(* Logix 5000 Rung export; software revision 16.04 *)

MODULES
   Local : vendor None type None code None
   MVI56E_AFC : vendor None type None code None
END_MODULES

TYPE AFCEComponents :   // High precision gas component analysis (only supported version 2.07.000)
STRUCT
   C1 : REAL;   // Methane
   N2 : REAL;   // Nitrogen
   CO2 : REAL;   // Carbon Dioxide
   C2 : REAL;   // Ethane
   C3 : REAL;   // Propane
   H20 : REAL;   // Water
   H2S : REAL;   // Hydrogen Sulphide
   H2 : REAL;   // Hydrogen
   CO : REAL;   // Carbon Monoxide
   O2 : REAL;   // Oxygen
   IC4 : REAL;   // Iso-butane
   NC4 : REAL;   // Normal Butane
   IC5 : REAL;   // Iso-pentane
   NC5 : REAL;   // Normal-pentane
   C6 : REAL;   // Hexane
   C7 : REAL;   // Heptane
   C8 : REAL;   // Octane
   C9 : REAL;   // Nonane
   C10 : REAL;   // Decane
   He : REAL;   // Helium
   Ar : REAL;   // Argon
   NeoC5 : REAL;   // Not Used
   UxUser1 : REAL;   // Not Used
   UyUser2 : REAL;   // Not Used
   UxUser3 : REAL;   // Not Used
   UyUser4 : REAL;   // Not Used
   UxUser5 : REAL;   // Not Used
   UyUser6 : REAL;   // Not Used
   UxUser7 : REAL;   // Not Used
   UyUser8 : REAL;   // Not Used
   UxUser9 : REAL;   // Not Used
   UyUser10 : REAL;   // Not Used
END_STRUCT
END_TYPE

TYPE AFCEMeterLinearGasProcess :   // Linear Gas Process Variables
STRUCT
   PulseFrequency : REAL;   // Pulse Frequency (Hz)
   Temperature : REAL;   // Temperature
   Pressure : REAL;   // Pressure
   MeterPulses : DINT;   // Pulse count
END_STRUCT
END_TYPE

TYPE AFCEProveProcess :   // Prove process output from processor to the module
STRUCT
   Sequencing : AFCEProveSequencing;   // Prover sequencing
   Temperature : REAL;   // Temperature for Single Probe provers. And Inlet Temperature for Dual Probe Provers.
   OutletTemperature : REAL;   // Outlet Temperature for Provers with Dual Probes.
   SwitchBarTemperature : REAL;   // Switch bar temperature
   Pressure : REAL;   // Pressure for Single Probe provers. And Inlet Pressure for Dual Probe Provers.
   OutletPressure : REAL;   // Outlet Pressure for Provers with Dual Probes.
   ProverDensity : REAL;   // Prover density
END_STRUCT
END_TYPE

TYPE AFCEMeterLinearGasArchiveFetch :
STRUCT
   Daily : AFCEMeterLinearGasArchiveFetchT;
   Hourly : AFCEMeterLinearGasArchiveFetchT;
END_STRUCT
END_TYPE

TYPE AFCEMeterControl :   // Enable/Disable Meter and Streams
STRUCT
   Meter : AFCEMeterControlMeter;   // Control the Meter
   Stream : AFCEMeterControlStream;   // Control the Meter Streams
   ResetAccumulators : AFCEMeterSignals;   // Resets for meter accumulators
END_STRUCT
END_TYPE

TYPE AFCEMeterLinearGasCalRequestProces :
STRUCT
   PulseFrequency : BOOL;   // Pulse Frequency
   Temperature : BOOL;   // Temperature
   Pressure : BOOL;   // Pressure
END_STRUCT
END_TYPE

TYPE AFCEModbusMasterDataType :   // Modbus master data type
STRUCT
   Bit : BOOL;   // bit type
   Word : BOOL;   // word type (16-bit)
   Long : BOOL;   // long integer (32-bit)
   LongRemote : BOOL;   // long integer (32-bit)
END_STRUCT
END_TYPE

TYPE AFCEProveSequencing :   // AFC prove sequencing tag for phase selection and ball positioning
STRUCT
   Phase : AFCEProvePhaseBitmap;   // AFC phase sequencing
   BallPositionReady : BOOL;   // Ball position: Ready (Udir & Bdir only; fwd leg Bdir)
   BallPositionSealed : BOOL;   // Ball position: Sealed (Udir & Bdir only; fwd leg Bdir)
   BallPositionReadyBwdLeg : BOOL;   // Ball position: Ready bwd leg (Bdir only)
   BallPositionSealedBwdLeg : BOOL;   // Ball position: Sealed bwd leg (Bdir only)
END_STRUCT
END_TYPE

TYPE AFCEUtil :   // Used for internal ladder logic usage. These values must not be changed by user application.
STRUCT
   Flags : AFCEFlag;   // Wallclock update commands
   CycleCounter : INT;   // Reflects current block ID calculated by ladder to be sent to the module
   Buffer : AFCEUtilBuffer;
   Block : AFCEUtilBlock;
END_STRUCT
END_TYPE

TYPE AFCEExtended :
STRUCT
   Trigger : BOOL;
   Data : AFCEExtendedData;
END_STRUCT
END_TYPE

TYPE AFCEMeterLinearGasBackPlaneReturn :   // Linear Gas Meter
STRUCT
   StandardDefault : AFCEMeterLinearGasStandardDflt;
   StandardRaw : INT[14];
   Extended : AFCEExtended;
END_STRUCT
END_TYPE

TYPE AFCEModbusGatewayCommand :   // Modbus Gateway Command
STRUCT
   Config : AFCEModbusGatewayConfig;   // Config data to be entered by the user.
   Trigger : BOOL;   // Trigger the Command, when cleared module has responded.
   Data : INT[200];   // Contains modbus data written to the module (write commands)
END_STRUCT
END_TYPE

TYPE AFCEMeterLinearGasArchiveFetchT :   // Fetch Archive
STRUCT
   Trigger : BOOL;   // Trigger Archive Fetch
   Age : INT;   // 0 = Current Archive
   Error : AFCEMeterArchiveFetchError;   // Archive Fetch Error
   Default : AFCEMeterLinearGasArchiveDflt;   // Default Archive
   Raw : INT[100];   // Raw Archive
END_STRUCT
END_TYPE

TYPE AFCEMeterStatusStream :
STRUCT
   Active : INT;   // Current Active Stream
   Enabled : AFCEMeterStatusStreamEnabled;   // Enabled Streams
   Configured : AFCEMeterStatusStreamEnabled;   // Configured Streams
   EnableAlarm : AFCEMeterStatusStreamAlarm;   // Enable Alarms
END_STRUCT
END_TYPE

TYPE AFCEProveRunResults :   // Run results of the prove. Copied from the module to the pocessor
STRUCT
   CountAttempted : INT;   // Run count attempted
   CountCompleted : INT;   // Run count completed
   CountSelected : INT;   // Run count selected
   RunsSelected : INT;   // Bit Mapped Runs selected for calculations from completed runs
   NewMeterFactor : REAL;   // New meter factor
   ChangeInMeterFactor : REAL;   // Change in meter factor
END_STRUCT
END_TYPE

TYPE AFCEModbusMasterSwap :   // Modbus master swap words/ swap bytes
STRUCT
   SwapWords : BOOL;   // Swap words
   SwapBytes : BOOL;   // Swap bytes
END_STRUCT
END_TYPE

TYPE AFCEModbusMaster :   // Modbus Master. Port 3 must be configured as modbus master through AFC Manager to use this feature.
STRUCT
   Enable : BOOL;   // Enable the modbus master funcionality
   CommandIndex : INT;   // Selects which command index will be executed
   Command : AFCEModbusMasterCommand[10];   // Each command contains a specific modbus request to be sent out of the port
END_STRUCT
END_TYPE

TYPE AFCEMeterLinearGasCalRequest :
STRUCT
   ProcessVariable : AFCEMeterLinearGasCalRequestProces;   // Process Variable
   ActionType : AFCEMeterCalRequestActionType;   // Action Type
   Value : AFCEMeterCalRequestActionValue;   // Value
   Count : DINT;   // Number of calibration requests
END_STRUCT
END_TYPE

TYPE AFCEMeterLinearGasArchiveDflt :   // Default Configuration
STRUCT
   ClosingTimestamp : DINT;
   CumulativeActiveStreams : INT;
   CurrentActiveStream : SINT;
   MeterStatus : SINT;
   FlowingPeriod : DINT;
   PeriodDuration : DINT;
   AccumulatorTotalizer : DINT;
   AccumulatorResidue : REAL;
   MeterAlarms : DINT;
   PulseFrequency : REAL;
   Temperature : REAL;
   Pressure : REAL;
   RelativeDensity : REAL;
   ReferenceCompressibility : REAL;
   FlowingCompressibility : REAL;
   Fpv : REAL;
   KFactor : REAL;
   MeterFactor : REAL;
   InputPulseCount : DINT;
   ManPulseCountCurrent : DINT;
   MassNRAccumulatorCurrent : REAL;   // Non-resettable
   MassNRAccumulatorOpening : REAL;   // Non-resettable
   EnergyNRAccumulatorCurrent : REAL;   // Non-resettable
   EnergyNRAccumulatorOpening : REAL;   // Non-resettable
   NetNRAccumulatorCurrent : REAL;   // Non-resettable
   NetNRAccumulatorOpening : REAL;   // Non-resettable
   GrossNRAccumulatorCurrent : REAL;   // Non-resettable
   GrossNRAccumulatorOpening : REAL;   // Non-resettable
   MolarFractionComponent01_C1 : REAL;
   MolarFractionComponent02_N2 : REAL;
   MolarFractionComponent03_CO2 : REAL;
   MolarFractionComponent04_C2 : REAL;
   MolarFractionComponent05_C3 : REAL;
   MolarFractionComponent06_H2O : REAL;
   MolarFractionComponent07_H2S : REAL;
   MolarFractionComponent08_H2 : REAL;
   MolarFractionComponent09_CO : REAL;
   MolarFractionComponent10_O2 : REAL;
   MolarFractionComponent11_IC4 : REAL;
   MolarFractionComponent12_NC4 : REAL;
   MolarFractionComponent13_IC5 : REAL;
   MolarFractionComponent14_NC5 : REAL;
   MolarFractionComponent15_C6 : REAL;
   MolarFractionComponent16_C7 : REAL;
   MolarFractionComponent17_C8 : REAL;
   MolarFractionComponent18_C9 : REAL;
   MolarFractionComponent19_C10 : REAL;
   MolarFractionComponent20_He : REAL;
   MolarFractionComponent21_Ar : REAL;
   UserSpecifiedFlowAverage1 : REAL;
   UserSpecifiedFlowAverage2 : REAL;
   UserSpecifiedFlowAverage3 : REAL;
END_STRUCT
END_TYPE

TYPE AFCEFlag :   // Flags contains status information updated by ladder and also trigger bits for clock update
STRUCT
   AFCStopped : BOOL;   // Indicates that the module has sent a new input block to be processed by ladder - UPDATED BY LADDER
   AFCInputSequenceNum : INT;   // Meter number (0 -15) associated to blocks 1-16. Used to update "Profile" (meter type and product group.) UPDATED BY LADDER
END_STRUCT
END_TYPE

TYPE AFCEModbusPassThruBitData :   // AFC Modbus Pass-thru Bit Data
STRUCT
   Data : BOOL[2016];   // Contains received data for bit commands
END_STRUCT
END_TYPE

TYPE AFCEUtilBlockInterrupt :
STRUCT
   Now : BOOL;
   ModbusGateway : DINT;
   EnableDisable : BOOL;
   Analysis : DINT;
END_STRUCT
END_TYPE

TYPE AFCEFirmwareVersion :
STRUCT
   Major : SINT;   // Major Version number
   Minor : SINT;   // Minor Version number
   Revision : INT;   // Revision
END_STRUCT
END_TYPE

TYPE AFCEModbusGateway :   // Modbus Gateway
STRUCT
   Command : AFCEModbusGatewayCommand[10];   // Modbus gateway commands - contains setup and modbus data
END_STRUCT
END_TYPE

TYPE AFCEMeterCalRequestActionType :
STRUCT
   ZeroShift : BOOL;   // Zero Shift
   SetZero : BOOL;   // Set Zero
   SetSpan : BOOL;   // Set Span
   SetMid1 : BOOL;   // Set Mid 1
   SetMid2 : BOOL;   // Set Mid 2
   SetMid3 : BOOL;   // Set Mid 3
END_STRUCT
END_TYPE

TYPE AFCEUtilBuffer :   // Buffer
STRUCT
   Input : INT[250];   // Input buffer contains the complete block to be copied from the module
   Output : INT[248];   // Output buffer contains data the complete block to be copied to the module
   Process : INT[240];
   ArchiveDay : INT[98];
   ArchiveHour : INT[98];
   Prove : INT[26];
   Analysis : INT[198];
   MeterEnableDisable : INT[4];
   StreamEnable : INT[48];
   StreamDisable : INT[48];
   StreamSelect : INT[32];
   MeterSignals : INT[32];
   Calibration : INT[36];
END_STRUCT
END_TYPE

TYPE AFCEUtilBlock :
STRUCT
   ProcessInput : INT;
   InterruptPending : AFCEUtilBlockInterrupt;
   InterruptComplete : AFCEUtilBlockInterrupt;
   NonInterruptPending : AFCEUtilBlockNonInterrupt;
   NonInterruptComplete : AFCEUtilBlockNonInterrupt;
END_STRUCT
END_TYPE

TYPE AFCEMeterSignals :   // Meter trigger accumulator and archive resets
STRUCT
   ResetAccumulator1 : BOOL;   // Set to 1 to reset resettable accumulator 1
   ResetAccumulator2 : BOOL;   // Set to 1 to reset resettable accumulator 2
   ResetAccumulator3 : BOOL;   // Set to 1 to reset resettable accumulator 3
   ResetAccumulator4 : BOOL;   // Set to 1 to reset resettable accumulator 4
END_STRUCT
END_TYPE

TYPE AFCEProve :   // Prove
STRUCT
   Process : AFCEProveProcess;   // Process Variables
   Signals : AFCEProveSignals;   // AFC Prove Signals (triggers the proving update)
   Config : AFCEProveConfig;   // AFC Prove Control (configuration settings)
   PulseCounts : AFCEProvePulseCount;   // Pulse counts to be updated at the end of the run/pass
   ConfigInput : AFCEProveInputConfig;   // AFC prover input configuration
   Status : AFCEProveStatus;   // AFC prover status
   ErrorCode : INT;   // Prove error code
   ProveControlsEcho : INT;   // AFC module Echos the state of the Prove Controls
   RequestedMeterEcho : INT;   // AFC module Echos the Meter number requested
   RequestedCurvePointEcho : INT;   // AFC module Echos the requested Curve Point
   RunResults : AFCEProveRunResults;   // Prove and run results
   ProveEnabled : BOOL;   // ON if prove is enabled. This flag is coped from inputbuffer[247]
END_STRUCT
END_TYPE

TYPE AFCEMeterControlStream :
STRUCT
   Selected : SINT;   // Stream to Enable or Disable and/or make active.
   EnableSelected : BOOL;   // Enable the Selected Stream
   DisableSelected : BOOL;   // Disable the Selected Stream
   SetSelectedToActive : BOOL;   // Set Selected to Active Stream
END_STRUCT
END_TYPE

TYPE AFCEProveConfig :   // Controls (configuration settings) associated to the prover
STRUCT
   Enable : AFCEProveConfigEnable;   // Controls at enable
   Accept : AFCEProveConfigAccept;   // Controls at accept
END_STRUCT
END_TYPE

TYPE AFCEWallclock :
STRUCT
   GetAFCTime : BOOL;   // Get current AFC Time
   SetAFCTimeFromPLCTime : BOOL;   // Set AFC time from PLC time. Updates current AFC time
   EnableLocalDateTime : BOOL;   // Enable Local Date Time.
   AFCTime : AFCETime;   // Coordinated Universal Time. Updated by either getting or setting AFC time.
END_STRUCT
END_TYPE

TYPE AFCEMeterCalRequestActionValue :
STRUCT
   ZeroShift : AFCEMeterCalRequestValue;   // Zero Shift
   SetZero : AFCEMeterCalRequestValue;   // Set Zero
   SetSpan : AFCEMeterCalRequestValue;   // Set Span
   SetMid1 : AFCEMeterCalRequestValue;   // Set Mid 1
   SetMid2 : AFCEMeterCalRequestValue;   // Set Mid 2
   SetMid3 : AFCEMeterCalRequestValue;   // Set Mid 3
END_STRUCT
END_TYPE

TYPE AFCEMeterStatus :   // Status
STRUCT
   Meter : AFCEMeterStatusMeter;   // Meter Status
   Stream : AFCEMeterStatusStream;   // Stream Status
END_STRUCT
END_TYPE

TYPE AFCEModbusMasterConfig :   // Modbus master command settings
STRUCT
   Enable : BOOL;   // Set to 1 to enable command (0=disable)
   FunctionType : BOOL;   // Set to 1 to select write command (0=read command)
   RegisterBank : BOOL;   // Set to 1 to select input register (0=holding register)
   DataType : AFCEModbusMasterDataType;   // Select data type format
   SwapOption : AFCEModbusMasterSwap;   // Select byte and word swap (1 = swap, 0 = no swap)
   TypeSwap : INT;   // This value is calculated by ladder logic and must not be modified by user
   SlaveAddress : INT;   // Modbus slave address of remote device
   ModbusAddress : INT;   // Modbus data address on remote slave
   ElementCount : INT;   // Number of data elements (125 words)
   TransactionID : INT;   // Transaction ID. This value is returned to the ReturnedTransaction ID when the response has been received.
END_STRUCT
END_TYPE

TYPE AFCEMeterStatusStreamEnabled :   // Stream Status 1 = Enabled
STRUCT
   Stream1 : BOOL;
   Stream2 : BOOL;
   Stream3 : BOOL;
   Stream4 : BOOL;
   Stream5 : BOOL;
   Stream6 : BOOL;
   Stream7 : BOOL;
   Stream8 : BOOL;
   Stream9 : BOOL;
   Stream10 : BOOL;
   Stream11 : BOOL;
   Stream12 : BOOL;
   Stream13 : BOOL;
   Stream14 : BOOL;
   Stream15 : BOOL;
   Stream16 : BOOL;
END_STRUCT
END_TYPE

TYPE AFCEMeterArchiveFetchError :
STRUCT
   ArchiveSelectionInvalid : BOOL;   // Archive File Selection Invalid
   AgeOutsideSize : BOOL;   // Age Outside Configured File Size
   ArchiveNeverWritten : BOOL;   // Age OK but Archive Record Never Written (new or reconfigured meter)
   Reserverd1 : BOOL;
   Reserverd2 : BOOL;
   Reserverd3 : BOOL;
   Reserverd4 : BOOL;
   Reserverd5 : BOOL;
   Reserverd6 : BOOL;
   Reserverd7 : BOOL;
   Reserverd8 : BOOL;
   Reserverd9 : BOOL;
   Reserverd10 : BOOL;
   Reserverd11 : BOOL;
   Reserverd12 : BOOL;
   Reserverd13 : BOOL;
END_STRUCT
END_TYPE

TYPE AFCESiteStatus :   // Site status bits - contains general information about the module - not meter specific
STRUCT
   AFCActive : BOOL;   // AFC active
   ChecksumAlarms : BOOL;   // Checkum alarm active
   Reserved2 : BOOL;
   Reserved3 : BOOL;
   PLCHalted : BOOL;   // PLC in program mode or missing
   CfgChanged : BOOL;   // Configuration changed
   Powerup : BOOL;   // Module powered up
   ColdStart : BOOL;   // Module performed cold start (BBRAM initialized)
   ModbusMasterPending : BOOL;   // Modbus Master Poll Pending
   ModbusMasterComplete : BOOL;   // Modbus Master Poll Complete
   ModbusPassThruPending : BOOL;   // Modbus Pass-thru Input Pending
   CalibrationRequest : BOOL;   // Calibration request from module
   ProverEnabled : BOOL;   // Prover Enabled
   Reserved13 : BOOL;
   Reserved14 : BOOL;
   Reserved15 : BOOL;
END_STRUCT
END_TYPE

TYPE AFCEMeterLinearGasArchive :   // Linear Gas Archive
STRUCT
   Write : AFCEMeterLinearGasArchiveWrite;
   Fetch : AFCEMeterLinearGasArchiveFetch;
END_STRUCT
END_TYPE

TYPE AFCEModuleDef :   // Main user defined data type
STRUCT
   ModbusGateway : AFCEModbusGateway;   // Reads and write data between processor and module modbus table
   ModbusMaster : AFCEModbusMaster;   // Setup modbus master commands to be sent to remote slaves (through Port 3)
   ModbusPassThru : AFCEModbusPassThru;   // Modbus pass-thru data
   SiteStatus : AFCESiteStatus;   // Site status
   MeterAlarms : AFCESiteAlarms;   // Meter Alarms
   Prove : AFCEProve;   // Prover
   Wallclock : AFCEWallclock;   // Set clock and get clock information
   Firmware : AFCEFirmwareVersion;   // Firmware information
   Util : AFCEUtil;   // Used by ladder logic
END_STRUCT
END_TYPE

TYPE AFCEModbusGatewayConfig :   // Modbus Ggateway Configuration
STRUCT
   Enable : BOOL;   // Set to 1 to enable modbus gateway command (0=disable)
   StartRegister : DINT;   // Start modbus address
   RegisterCount : INT;   // Word count (200 max)
   FunctionType : BOOL;   // 0 = read command, 1 = write command
   RegisterType : BOOL;   // 0 = holding register, 1 = input register
   SlaveType : BOOL;   // 0 = primary slave, 1 = virtual slave
END_STRUCT
END_TYPE

TYPE AFCEMeterLinearGasAlarm :
STRUCT
   Control : AFCEMeterLinearGasAlarmControl;   // Alarm Control
END_STRUCT
END_TYPE

TYPE AFCEMeterCalRequestValue :
STRUCT
   Applied : REAL;   // Applied
   Measured : REAL;   // Measured
END_STRUCT
END_TYPE

TYPE AFCEMeterProcessAlarmFidelity :   // Process Alarms
STRUCT
   SetGeneralFail : BOOL;   // Set to indicate General Failure of the Transmitter
   StaleData : BOOL;   // Clear to Indicate new process input data
   Reserved : BOOL;   // Reserved
   SetPulseFidelityAlarm : BOOL;   // Set to indicate Pulse Fidelity Alarm
   SetAutoClearStaleData : BOOL;   // Set to automatically clear stale data
END_STRUCT
END_TYPE

TYPE AFCEMeterLinearGasAlarmControl :   // Linear Gas Process Alarms
STRUCT
   PulseFrequency : AFCEMeterProcessAlarm;   // Pulse Frequency Alarms
   Temperature : AFCEMeterProcessAlarm;   // Temperature Alarms
   Pressure : AFCEMeterProcessAlarm;   // Pressure Alarms
   MeterPulses : AFCEMeterProcessAlarmFidelity;   // Meter Pulses Alarms
END_STRUCT
END_TYPE

TYPE AFCEUtilBlockNonInterrupt :
STRUCT
   Now : BOOL;
   ModbusMasterCommand : BOOL;
   ModbusMasterResponse : BOOL;
   Archive : DINT;
   Prover : BOOL;
   PassThru : BOOL;
   Calibration : BOOL;
END_STRUCT
END_TYPE

TYPE AFCEProveConfigAccept :   // Prove controls at accept. If auto-accept is selected must be available at enable
STRUCT
   RequestedInterpolationPoint : INT;   // Requested interpolation point (0 nearest)
   ApplyMFChangeAllStreams : BOOL;   // Apply change in meter factor to all streams
   ApplyMFChangeCurve : BOOL;   // Apply change in meter factor to all curve points
   ApplyNewMF : BOOL;   // CApply new meter factor
END_STRUCT
END_TYPE

TYPE AFCEProvePhaseBitmap :   // AFC prove phase bitmap
STRUCT
   NotSelected : BOOL;   // Not selected
   Active : BOOL;   // Active, not counting
   CountingPast1stSwitch : BOOL;   // Counting past 1st switch for Udir and forward leg for Bdir)
   Past2ndSwitchFwdLeg : BOOL;   // Past 2nd switch forward leg (bidirectional only)
   Past1stSwithRetLeg : BOOL;   // Past 1st switch return leg (bidirectional only)
   RunComplete : BOOL;   // Run complete. past 2nd switch.
END_STRUCT
END_TYPE

TYPE AFCETime :   // AFC time format used for wallclock update.
STRUCT
   Year : DINT;   // Year
   Month : DINT;   // Month
   Day : DINT;   // Day
   Hour : DINT;   // Hour
   Minute : DINT;   // Minute
   second : DINT;   // Seconds
END_STRUCT
END_TYPE

TYPE AFCEProveSignals :   // Contains the proving signals that will trigger specific tasks from the module
STRUCT
   EnableProve : BOOL;   // Enables the prove
   AcceptProve : BOOL;   // Accepts the prove
   RejectProve : BOOL;   // Reject the prove
   RunStart : BOOL;   // Starts the run
   RunComplete : BOOL;   // Flags that the run is complete
   RunCancel : BOOL;   // Cancels the run
   RunDelete : BOOL;   // Deletes the run
   PassComplete : BOOL;   // Flag that the pass is complete
   PauseProve : BOOL;   // Pauses the Proving Process
   AbortProve : BOOL;   // Aborts the prove
END_STRUCT
END_TYPE

TYPE AFCEMeterProfile :   // Meter configuration profile
STRUCT
   MeterType : BOOL;   // 0=Differential, 1=Linear
   ProductGroup : BOOL;   // 0=Gas, 1=Liquid
   PrimaryInput : BOOL;   // For differential, 0=Differential Pressure 1=Flow Rate. For Linear, 0=Pulse Count 1=Pulse Frequency
   AOIMismatch : BOOL;   // AOI Meter type does not match module for meter number
END_STRUCT
END_TYPE

TYPE AFCEMeterStatusStreamAlarm :   // Stream Alarms
STRUCT
   StreamOutOfRange : BOOL;   // Requested Stream Number Out of Range
   StreamNotConfigured : BOOL;   // Requested Stream not Configured
   StreamNotEnabled : BOOL;   // Requested Stream not Enabled
   EventLogFull : BOOL;   // Event Log Full, Action not Performed
END_STRUCT
END_TYPE

TYPE AFCEModbusPassThru :   // AFC Modbus Pass-thru
STRUCT
   Enable : BOOL;   // Set to 1 to enable pass-thru functionality (requires AFC Manager setting)
   MessagePresent : BOOL;   // Message present in the response block
   GetMessage : BOOL;   // Get the pass-thru message. When the bit is cleared the message has been transferred to the PLC.
   FunctionBitWrite : BOOL;   // Function bit write
   OverflowError : BOOL;   // Overflow error flag
   ModbusAddress : INT;   // Destination modbus address
   RegisterCount : INT;   // Number of elements associated to command
   ReadDataWord : INT[125];   // Contains received data for word commands
   ReadDataBit : AFCEModbusPassThruBitData;   // Contains received data for bit commands
END_STRUCT
END_TYPE

TYPE AFCEProveInputConfig :   // Prove input block results - prover configuration
STRUCT
   Type : INT;   // Prover type
   Options : INT;   // Prover options
   RunsPerProveTotal : INT;   // Total runs per prove
   RunsPerProveSelected : INT;   // Selected runs per prove
   MaxRunsBeforeAbort : INT;   // Max total runs before abort
   ShortPassesPerRun : INT;   // Short passes per run if bidir = 2 , else 0
END_STRUCT
END_TYPE

TYPE AFCEMeterLinearGas :   // Linear Gas Meter
STRUCT
   Control : AFCEMeterControl;   // Meter Control
   Status : AFCEMeterStatus;   // Meter Status
   ProcessVariables : AFCEMeterLinearGasProcess;   // Input process variables to be transferred to the module
   Analysis : AFCEMeterAnalysis;   // Molar Analysis data to be transferred to the module (only for gas products with online gas chromatograph applications)
   Alarm : AFCEMeterLinearGasAlarm;   // Meter Alarms
   Archive : AFCEMeterLinearGasArchive;   // Archive
   Profile : AFCEMeterProfile;   // Module profile (meter type/product group) transfered from the module
   Calibration : AFCEMeterLinearGasCal;   // Calibration
   BackPlaneReturn : AFCEMeterLinearGasBackPlaneReturn;
END_STRUCT
END_TYPE

TYPE AFCEProveStatus :   // Status of the prove (returned from the module to the processor)
STRUCT
   ProveAccepted : BOOL;   // Prove was accepted
   MeterFactorApplied : BOOL;   // Meter factor was applied
   MFAppliedToCurve : BOOL;   // Meter factor was applied to all points in the curve
   MFAppliedToStreams : BOOL;   // Meter factor was applied to all streams
   ProveRejectedByCommand : BOOL;   // Prove was rejected by command
   ProveRejectedNoRuns : BOOL;   // Prove was rejected - empty prove (no runs)
   ProveRejectedDivideBy0 : BOOL;   // Prove was rejected - divide by 0
   ProveEnabled : BOOL;   // Prove is enabled
   ProvingRunInProgress : BOOL;   // Proving run is in progress
   ProveRejectedAbort : BOOL;   // Prove rejected: abort
   ProvePaused : BOOL;   // Prove is paused
   RunCancelled : BOOL;   // Run Is cancelled
   RunTimedOut : BOOL;   // Run timed out
END_STRUCT
END_TYPE

TYPE AFCEMeterProcessAlarm :   // Process Alarms
STRUCT
   SetGeneralFail : BOOL;   // Set to indicate General Failure of the Transmitter
   StaleData : BOOL;   // Clear to Indicate new process input data
   SetLowThreshold : BOOL;   // Set to indicate Lower Range Limit Exceeded
   SetHighThreshold : BOOL;   // Set to indicate Upper Range Limit Exceeded
   SetAutoClearStaleData : BOOL;   // Set to automatically clear stale data
END_STRUCT
END_TYPE

TYPE AFCEProveConfigEnable :   // Prove controls at enable
STRUCT
   MeterNumber : INT;   // Meter number requested (1-16)
   AutoAcceptProve : BOOL;   // Auto-accept the prove
   AutoContinueProve : BOOL;   // Auto-continue the prove
END_STRUCT
END_TYPE

TYPE AFCEMeterLinearGasStandardDflt :   // Linear Gas Meter Default Standard Data
STRUCT
   Meter_Alarms : DINT;   // Meter alarms
   NR_Acc_Net_Totalizer : DINT;   // Non-resettable accumulator, net, totalizer (m3)
   NR_Acc_Net_Residue : REAL;   // Non-resettable accumulator, net, residue (m3)
   FlowRate_Net : REAL;   // Flow rate, net (m3/h)
   FlowRate_Gross : REAL;   // Flow rate, gross / indicated (m3/h)
   Ifpv : REAL;   // AGA 8, Supercompressibility, Fpv
   Cprime : REAL;   // C-prime
END_STRUCT
END_TYPE

TYPE AFCEMeterAnalysis :   // Meter analysis components. Allows the processor to update molar analysis for low precision and high precision streams.
STRUCT
   Trigger : BOOL;   // Set to 1 to Send Updated Component Data to the Module
   Stream : INT;   // Stream for Analysis. Select 0 for current active stream.
   Error : AFCEMeterAnalysisError;   // Analysis Error
   Components : AFCEComponents;   // High precision gas components (floating point per component). Only supported for firmware version 2.07.000 or later
END_STRUCT
END_TYPE

TYPE AFCEMeterStatusMeter :   // Meter Status
STRUCT
   Enabled : BOOL;   // Meter Enable Status, 1=enabled
   EnableAlarm : BOOL;   // If set either: 1. The meter is not configured. 2. The event log is full, the action was not performed.
END_STRUCT
END_TYPE

TYPE AFCEMeterControlMeter :   // Enable and Disable Meter
STRUCT
   Enable : BOOL;   // Enable the Meter
   Disable : BOOL;   // Disable the Meter
END_STRUCT
END_TYPE

TYPE AFCEModbusMasterCommand :   // Modbus Master Command
STRUCT
   Config : AFCEModbusMasterConfig;   // Modbus Master Configuration
   ErrorCode : INT;   // Error Code associated to Modbus Master Command
   Pending : BOOL;   // Pending Modbus Master Command - waiting for Modbus Response
   ReturnedTransactionID : DINT;   // Changes to Config.TransactionID value when response has returned.
   Data : INT[100];   // Read or Write Data
END_STRUCT
END_TYPE

TYPE AFCEMeterLinearGasArchiveWrite :   // Write Archive
STRUCT
   Daily : BOOL;   // Set to 1 to write daily archive
   Hourly : BOOL;   // Set to 1 to write hourly archive
END_STRUCT
END_TYPE

TYPE AFCEProvePulseCount :   // Values to be supplied at the end of the pass/run
STRUCT
   Meter : DINT;   // Meter pulse count
   MasterMeter : DINT;   // Master meter pulse count
END_STRUCT
END_TYPE

TYPE AFCEMeterLinearGasCal :   // Processor Mediated Calibration
STRUCT
   Request : AFCEMeterLinearGasCalRequest;   // Calibration Request from module
   Response : AFCEMeterCalResponse;   // Processor Response
END_STRUCT
END_TYPE

TYPE AFCEMeterCalResponse :
STRUCT
   Trigger : BOOL;   // Send Error Code and Values to module to be recorded
   ErrorCode : SINT;   // Error Code to send. 0-4 allowed. 0=No error. 1-4=User defined.
   Value : AFCEMeterCalRequestValue;   // Value to Send
   Count : DINT;   // Number of calibration responses
END_STRUCT
END_TYPE

TYPE AFCEExtendedData :
STRUCT
   Raw : INT[64];
END_STRUCT
END_TYPE

TYPE AFCESiteAlarms :   // Indicates if a meter has any alarms
STRUCT
   Meter1 : BOOL;   // Meter in alarm
   Meter2 : BOOL;   // Meter in alarm
   Meter3 : BOOL;   // Meter in alarm
   Meter4 : BOOL;   // Meter in alarm
   Meter5 : BOOL;   // Meter in alarm
   Meter6 : BOOL;   // Meter in alarm
   Meter7 : BOOL;   // Meter in alarm
   Meter8 : BOOL;   // Meter in alarm
   Meter9 : BOOL;   // Meter in alarm
   Meter10 : BOOL;   // Meter in alarm
   Meter11 : BOOL;   // Meter in alarm
   Meter12 : BOOL;   // Meter in alarm
   Meter13 : BOOL;   // Meter in alarm
   Meter14 : BOOL;   // Meter in alarm
   Meter15 : BOOL;   // Meter in alarm
   Meter16 : BOOL;   // Meter in alarm
END_STRUCT
END_TYPE

TYPE AFCEMeterAnalysisError :
STRUCT
   StreamOutOfRange : BOOL;   // Requested Stream Number Out of Range
   StreamNotConfigured : BOOL;   // Requested Stream Not Configured
END_STRUCT
END_TYPE

ADD_ON_INSTRUCTION AOI56EAFCMeterLinearGas   (* revision 1.8, vendor ProSoft Technology Inc., ExecutePrescan *)
// Add-On instruction for the MVI56E-AFC.
// Linear Gas Meter
// Revision note:
// Corrected/Reverted ProcessInputBlockID Tag Data Type from INT to DINT.
// Help:
// Compatible with version 4.03 of MVI56E-AFC firmware or higher.
// v1.2: Remove Calculation Results. Add Backplane Return. Add Stale Data
// v1.3: Corrected an bug On Rung 2 for Linear Gas Meter AOI ProfileBuffer[0].4 for AOIMismatch.
// v1.4: Addition of default process input backplane return data mapping.
// v1.5: Made correlation changes between the Module Archive Default UDTs and the AOI Archive Default UDTs.
// v1.6: Made changes to the ModbusGatewayConfig UDT StartRegister Tag Data Type from INT to DINT
// and Modified ProcessInputBlockID Tag Data Type from DINT to INT.
// v1.7: Updated Tags names AFCMeterXXYYYYYY.BackPlaneReturn.ProcessInputs to
// AFCMeterXXYYYYYY.BackPlaneReturn.Standard and
// AFCMeterXXYYYYYY.BackPlaneReturn.ComponentAnalysis
//  to AFCMeterXXYYYYYY.BackPlaneReturn.Extended
// v1.8:  Corrected/Reverted ProcessInputBlockID Tag Data Type from INT to DINT.
VAR_IN_OUT
   ConnectionInput : INT[250]; {required}
   AFC : AFCEModuleDef; {required}
   AFCMeter : AFCEMeterLinearGas; {required}
END_VAR
VAR_INPUT
   MeterNumber : SINT; {required}   // Meter Number Set to a number between 1 and 16
END_VAR
VAR
   StreamSelectedShift : DINT;
   StreamSelectBuffer : INT;
   EnabledStatusBuffer : INT;
   StreamSelectBlockID : DINT;
   StreamNumberShift : DINT;
   StreamErrorBuffer : DINT;
   StreamEnableBlockID : DINT;
   StreamEnableBitPosition : DINT;
   StreamDisableBlockID : DINT;
   ProfileBuffer : SINT[2];
   ProcessInputBlockID : DINT;
   AnalysisGroupBitPosition : INT;
   AnalysisErrorBuffer : INT;
   ProcessAlarmShifter : DINT;
   ProcessAlarmBuffer : DINT;
   MeterSignaltBlockID : DINT;
   MeterNumberShift : DINT;
   MeterNumberBitPostition : DINT;
   Inputbuffer : INT[250];
   CalibrationMeterNumberBuffer : DINT;
   CalibrationMediationPending : BOOL;
   CalibrationInputScalingIndex : DINT;
   CalibrationHandleBuffer : DINT;
   ArchiveStream : DINT;
   ArchiveMeterStatusRaw : DINT;
   ArchiveMeterStatusActiveStream : DINT;
   ArchiveCompleteBitCheck : DINT;
   ArchiveBlockID : DINT;
   AnalysisGroupShift : DINT;
   AnalysisCompleteBitCheck : DINT;
   AnalysisBufferOffset : DINT;
   AnalysisBlockID : DINT;
   AFCStopped : BOOL;
   AFCInputDataAvailable : BOOL;
END_VAR

ROUTINE Logic   (* ladder *)
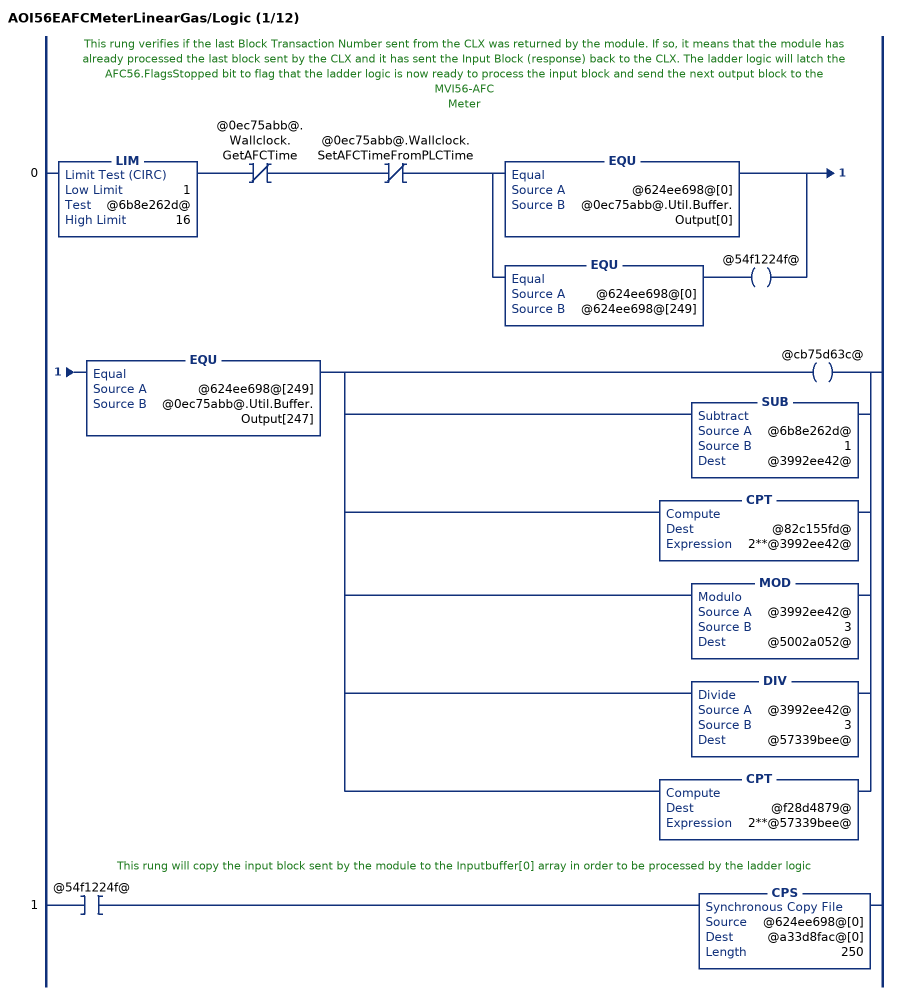
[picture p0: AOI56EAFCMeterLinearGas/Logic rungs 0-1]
   // This rung verifies if the last Block Transaction Number sent from the CLX was returned by the module. If so, it means that the module has already processed the last block sent by the CLX and it has sent the Input Block (response) back to the CLX. The ladder logic will latch the AFC56.FlagsStopped bit to flag that the ladder logic is now ready to process the input block and send the next output block to the MVI56-AFC
   // Meter
   0: LIM(1,@6b8e262d@,16)XIO(@0ec75abb@.Wallclock.GetAFCTime)XIO(@0ec75abb@.Wallclock.SetAFCTimeFromPLCTime)[EQU(@624ee698@[0],@0ec75abb@.Util.Buffer.Output[0]) ,EQU(@624ee698@[0],@624ee698@[249]) OTE(@54f1224f@) ]EQU(@624ee698@[249],@0ec75abb@.Util.Buffer.Output[247])[OTE(@cb75d63c@) ,SUB(@6b8e262d@,1,@3992ee42@) ,CPT(@82c155fd@,2**@3992ee42@) ,MOD(@3992ee42@,3,@5002a052@) ,DIV(@3992ee42@,3,@57339bee@) ,CPT(@f28d4879@,2**@57339bee@) ];
   // This rung will copy the input block sent by the module to the Inputbuffer[0] array in order to be processed by the ladder logic
   1: XIC(@54f1224f@)CPS(@624ee698@[0],@a33d8fac@[0],250);
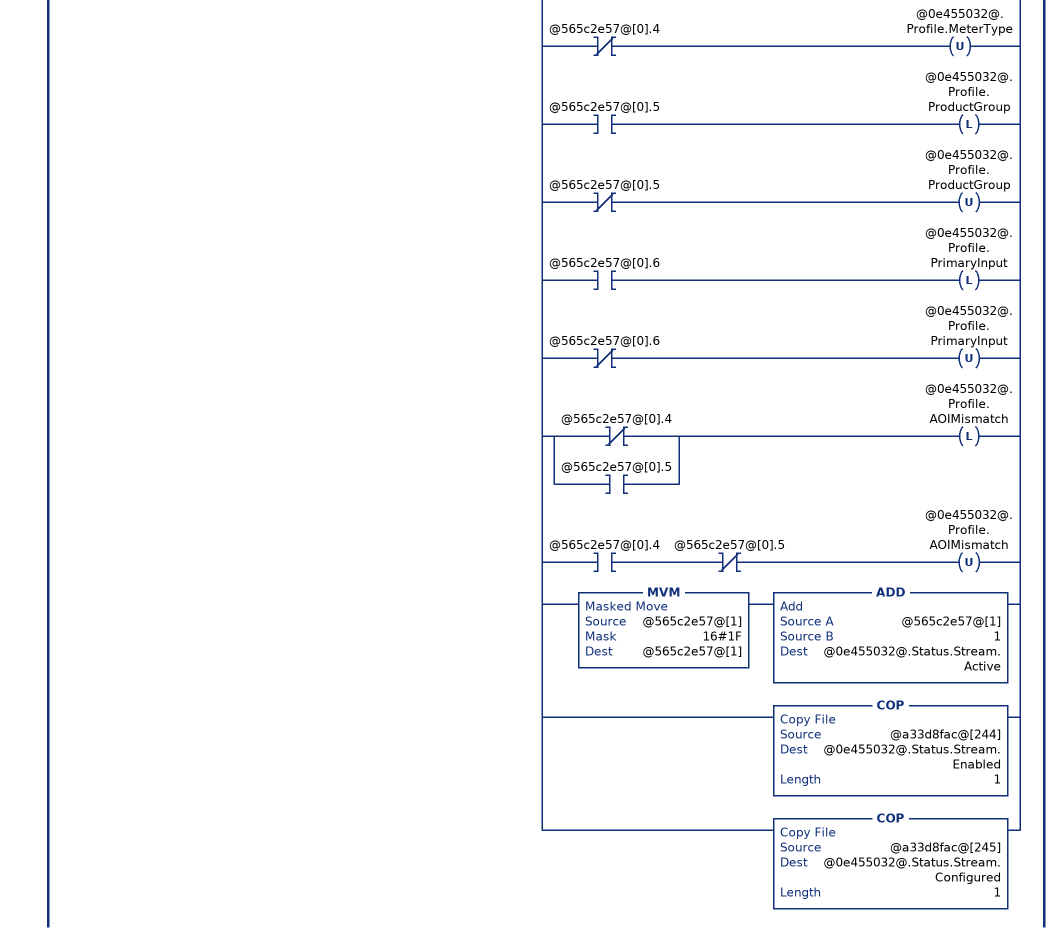
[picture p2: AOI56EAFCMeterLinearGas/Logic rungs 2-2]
   // Read process input backplane return and
   // meter profile (when block ID matches meter number).
   2: XIC(@54f1224f@)LIM(1,@a33d8fac@[0],16)[COP(@a33d8fac@[3+@3992ee42@*15],@0e455032@.BackPlaneReturn.StandardRaw[0],14) ,COP(@0e455032@.BackPlaneReturn.StandardRaw[0],@0e455032@.BackPlaneReturn.StandardDefault,1) ,COP(@a33d8fac@[247],@0ec75abb@.SiteStatus,1) ,COP(@a33d8fac@[248],@0ec75abb@.MeterAlarms,1) ,EQU(@a33d8fac@[0],@6b8e262d@) [COP(@a33d8fac@[243],@565c2e57@[0],2) ,[XIC(@565c2e57@[0].0) OTL(@0e455032@.Status.Meter.EnableAlarm) ,XIO(@565c2e57@[0].0) OTU(@0e455032@.Status.Meter.EnableAlarm) ] ,[XIC(@565c2e57@[0].1) OTL(@0e455032@.Status.Meter.Enabled) ,XIO(@565c2e57@[0].1) OTU(@0e455032@.Status.Meter.Enabled) ] ,[[XIC(@565c2e57@[0].4) OTL(@0e455032@.Profile.MeterType) ,XIO(@565c2e57@[0].4) OTU(@0e455032@.Profile.MeterType) ] ,[XIC(@565c2e57@[0].5) OTL(@0e455032@.Profile.ProductGroup) ,XIO(@565c2e57@[0].5) OTU(@0e455032@.Profile.ProductGroup) ] ,[XIC(@565c2e57@[0].6) OTL(@0e455032@.Profile.PrimaryInput) ,XIO(@565c2e57@[0].6) OTU(@0e455032@.Profile.PrimaryInput) ] ] ,[[XIO(@565c2e57@[0].4) ,XIC(@565c2e57@[0].5) ] OTL(@0e455032@.Profile.AOIMismatch) ,XIC(@565c2e57@[0].4) XIO(@565c2e57@[0].5) OTU(@0e455032@.Profile.AOIMismatch) ] ,MVM(@565c2e57@[1],16#1F,@565c2e57@[1]) ADD(@565c2e57@[1],1,@0e455032@.Status.Stream.Active) ,COP(@a33d8fac@[244],@0e455032@.Status.Stream.Enabled,1) ,COP(@a33d8fac@[245],@0e455032@.Status.Stream.Configured,1) ] ];
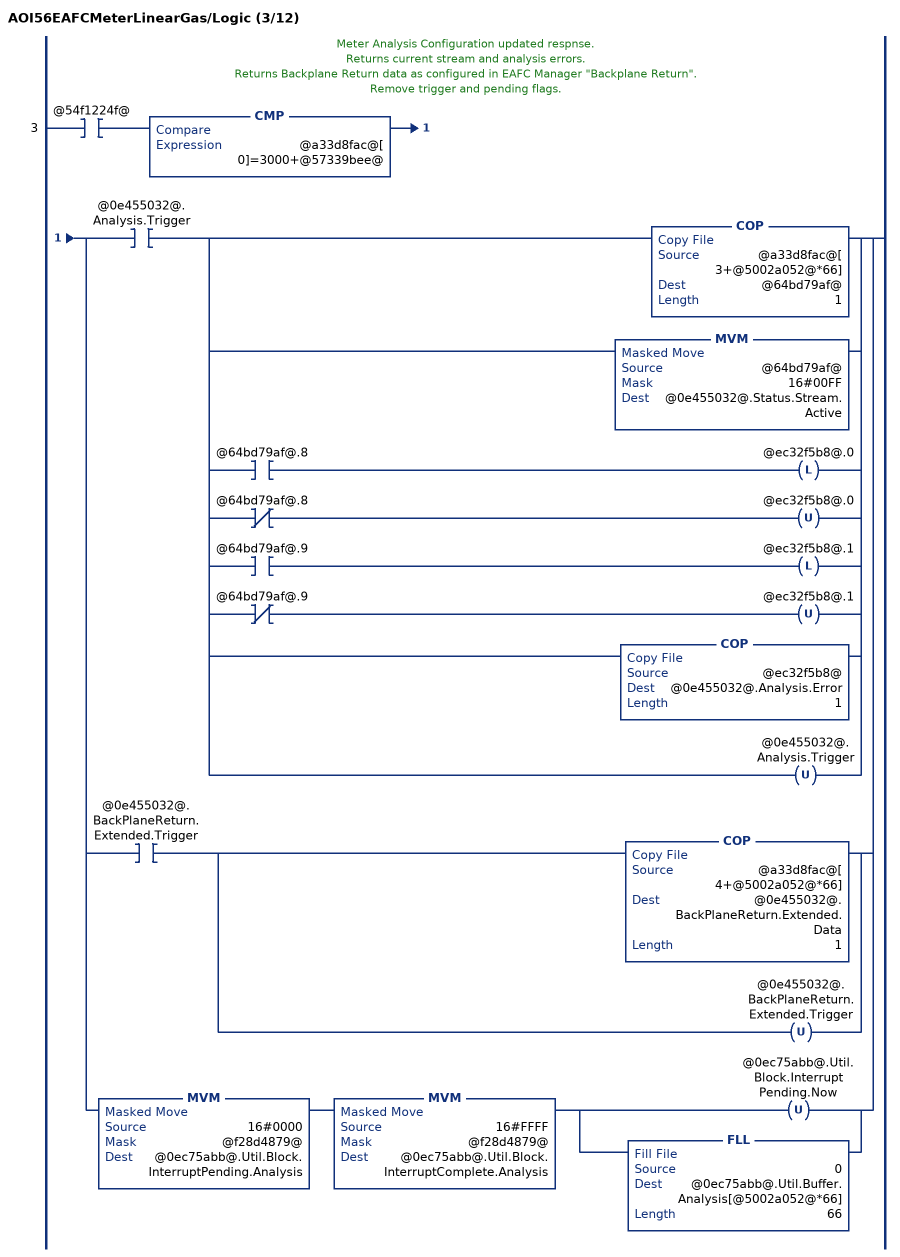
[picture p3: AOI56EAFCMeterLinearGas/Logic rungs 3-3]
   // Meter Analysis Configuration updated respnse.
   // Returns current stream and analysis errors.
   // Returns Backplane Return data as configured in EAFC Manager "Backplane Return".
   // Remove trigger and pending flags.
   3: XIC(@54f1224f@)CMP(@a33d8fac@[0]=3000+@57339bee@)[XIC(@0e455032@.Analysis.Trigger) [COP(@a33d8fac@[3+@5002a052@*66],@64bd79af@,1) ,MVM(@64bd79af@,16#00FF,@0e455032@.Status.Stream.Active) ,[XIC(@64bd79af@.8) OTL(@ec32f5b8@.0) ,XIO(@64bd79af@.8) OTU(@ec32f5b8@.0) ] ,[XIC(@64bd79af@.9) OTL(@ec32f5b8@.1) ,XIO(@64bd79af@.9) OTU(@ec32f5b8@.1) ] ,COP(@ec32f5b8@,@0e455032@.Analysis.Error,1) ,OTU(@0e455032@.Analysis.Trigger) ] ,XIC(@0e455032@.BackPlaneReturn.Extended.Trigger) [COP(@a33d8fac@[4+@5002a052@*66],@0e455032@.BackPlaneReturn.Extended.Data,1) ,OTU(@0e455032@.BackPlaneReturn.Extended.Trigger) ] ,MVM(16#0000,@f28d4879@,@0ec75abb@.Util.Block.InterruptPending.Analysis) MVM(16#FFFF,@f28d4879@,@0ec75abb@.Util.Block.InterruptComplete.Analysis) [OTU(@0ec75abb@.Util.Block.InterruptPending.Now) ,FLL(0,@0ec75abb@.Util.Buffer.Analysis[@5002a052@*66],66) ] ];
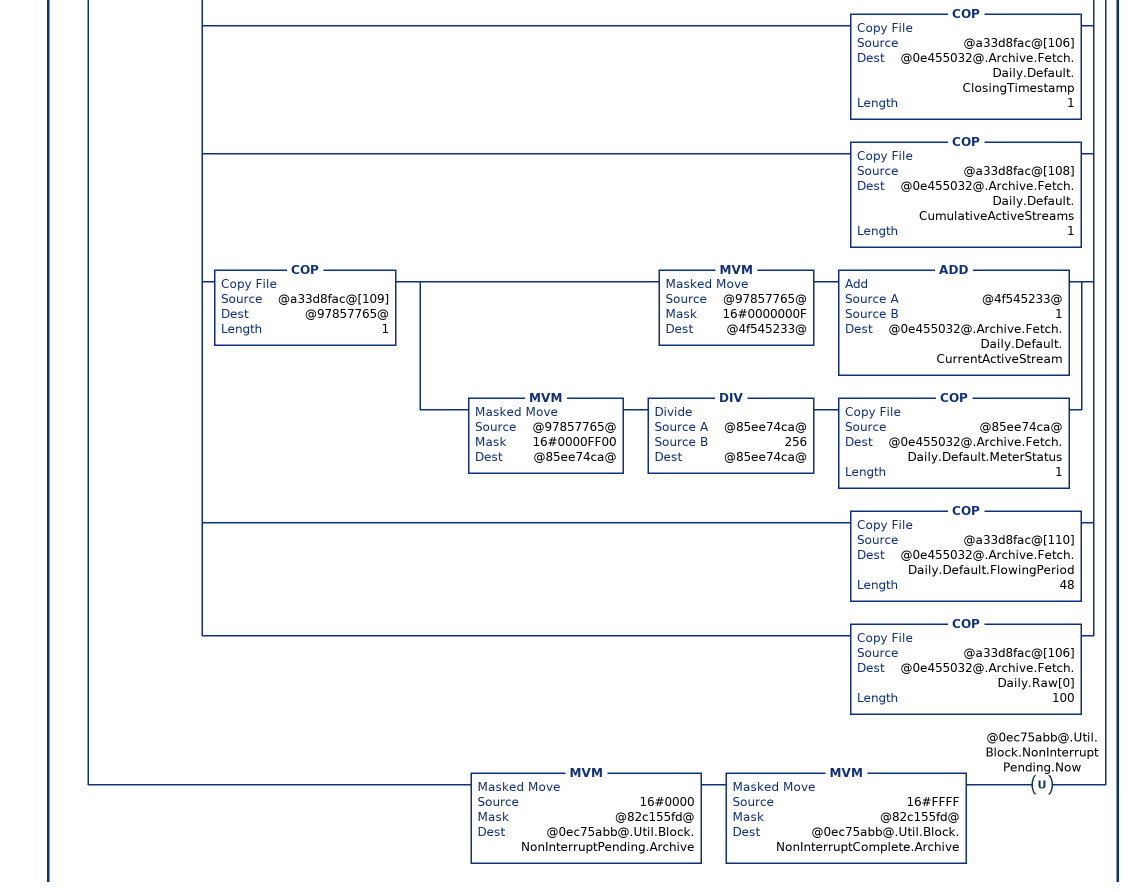
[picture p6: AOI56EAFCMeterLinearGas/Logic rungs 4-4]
   // Archive Fetch to default and raw UDT's.
   // Get archive alarms.
   // Remove trigger and pending flags.
   4: XIC(@54f1224f@)CMP(@a33d8fac@[0]=6000+@3992ee42@)[XIC(@0e455032@.Archive.Fetch.Hourly.Trigger) [OTU(@0e455032@.Archive.Fetch.Hourly.Trigger) ,[[XIC(@a33d8fac@[3].0) OTL(@0e455032@.Archive.Fetch.Hourly.Error.ArchiveSelectionInvalid) ,XIO(@a33d8fac@[3].0) OTU(@0e455032@.Archive.Fetch.Hourly.Error.ArchiveSelectionInvalid) ] ,[XIC(@a33d8fac@[3].1) OTL(@0e455032@.Archive.Fetch.Hourly.Error.AgeOutsideSize) ,XIO(@a33d8fac@[3].1) OTU(@0e455032@.Archive.Fetch.Hourly.Error.AgeOutsideSize) ] ,[XIC(@a33d8fac@[3].2) OTL(@0e455032@.Archive.Fetch.Hourly.Error.ArchiveNeverWritten) ,XIO(@a33d8fac@[3].2) OTU(@0e455032@.Archive.Fetch.Hourly.Error.ArchiveNeverWritten) ] ] ,COP(@a33d8fac@[4],@0e455032@.Archive.Fetch.Hourly.Default.ClosingTimestamp,1) ,COP(@a33d8fac@[6],@0e455032@.Archive.Fetch.Hourly.Default.CumulativeActiveStreams,1) ,COP(@a33d8fac@[7],@97857765@,1) [MVM(@97857765@,16#0000000F,@4f545233@) ADD(@4f545233@,1,@0e455032@.Archive.Fetch.Hourly.Default.CurrentActiveStream) ,MVM(@97857765@,16#0000FF00,@85ee74ca@) DIV(@85ee74ca@,256,@85ee74ca@) COP(@85ee74ca@,@0e455032@.Archive.Fetch.Hourly.Default.MeterStatus,1) ] ,COP(@a33d8fac@[8],@0e455032@.Archive.Fetch.Hourly.Default.FlowingPeriod,48) ,COP(@a33d8fac@[4],@0e455032@.Archive.Fetch.Hourly.Raw[0],100) ] ,XIC(@0e455032@.Archive.Fetch.Daily.Trigger) [OTU(@0e455032@.Archive.Fetch.Daily.Trigger) ,[[XIC(@a33d8fac@[105].0) OTL(@0e455032@.Archive.Fetch.Daily.Error.ArchiveSelectionInvalid) ,XIO(@a33d8fac@[105].0) OTU(@0e455032@.Archive.Fetch.Daily.Error.ArchiveSelectionInvalid) ] ,[XIC(@a33d8fac@[105].1) OTL(@0e455032@.Archive.Fetch.Daily.Error.AgeOutsideSize) ,XIO(@a33d8fac@[105].1) OTU(@0e455032@.Archive.Fetch.Daily.Error.AgeOutsideSize) ] ,[XIC(@a33d8fac@[105].2) OTL(@0e455032@.Archive.Fetch.Daily.Error.ArchiveNeverWritten) ,XIO(@a33d8fac@[105].2) OTU(@0e455032@.Archive.Fetch.Daily.Error.ArchiveNeverWritten) ] ] ,COP(@a33d8fac@[106],@0e455032@.Archive.Fetch.Daily.Default.ClosingTimestamp,1) ,COP(@a33d8fac@[108],@0e455032@.Archive.Fetch.Daily.Default.CumulativeActiveStreams,1) ,COP(@a33d8fac@[109],@97857765@,1) [MVM(@97857765@,16#0000000F,@4f545233@) ADD(@4f545233@,1,@0e455032@.Archive.Fetch.Daily.Default.CurrentActiveStream) ,MVM(@97857765@,16#0000FF00,@85ee74ca@) DIV(@85ee74ca@,256,@85ee74ca@) COP(@85ee74ca@,@0e455032@.Archive.Fetch.Daily.Default.MeterStatus,1) ] ,COP(@a33d8fac@[110],@0e455032@.Archive.Fetch.Daily.Default.FlowingPeriod,48) ,COP(@a33d8fac@[106],@0e455032@.Archive.Fetch.Daily.Raw[0],100) ] ,MVM(16#0000,@82c155fd@,@0ec75abb@.Util.Block.NonInterruptPending.Archive) MVM(16#FFFF,@82c155fd@,@0ec75abb@.Util.Block.NonInterruptComplete.Archive) OTU(@0ec75abb@.Util.Block.NonInterruptPending.Now) ];
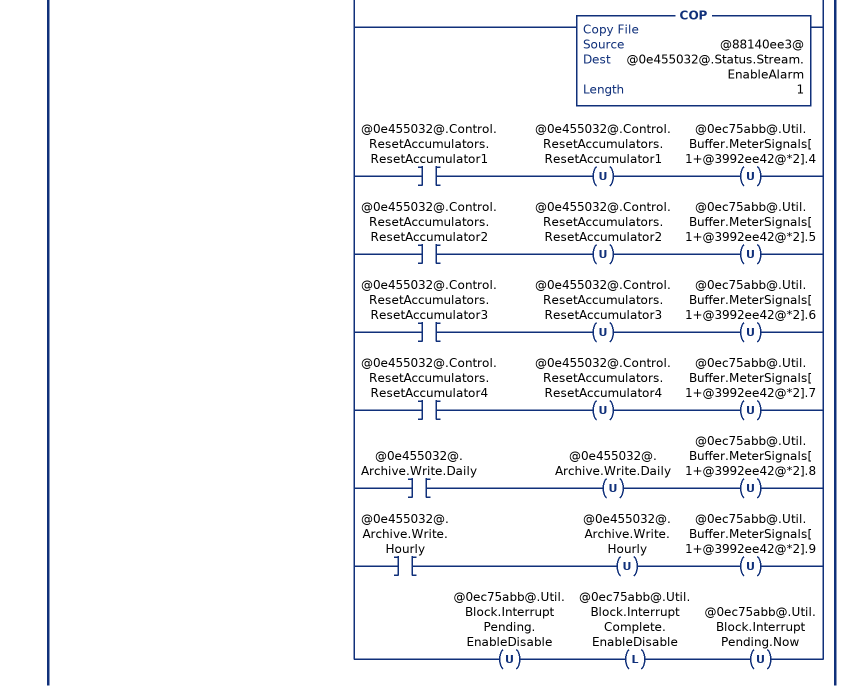
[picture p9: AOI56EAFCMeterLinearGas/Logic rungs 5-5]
   // Meter status and stream status.
   // Remove trigger and pending flags.
   5: XIC(@54f1224f@)EQU(@a33d8fac@[0],7000)[[MVM(@a33d8fac@[3],@82c155fd@,@7c715bd6@) ,[NEQ(@7c715bd6@,0) OTL(@0e455032@.Status.Meter.Enabled) ,EQU(@7c715bd6@,0) OTU(@0e455032@.Status.Meter.Enabled) ] ,OTU(@0e455032@.Control.Meter.Enable) MVM(16#0000,@82c155fd@,@0ec75abb@.Util.Buffer.MeterEnableDisable[1]) ,OTU(@0e455032@.Control.Meter.Disable) MVM(16#0000,@82c155fd@,@0ec75abb@.Util.Buffer.MeterEnableDisable[3]) ] ,[XIC(@0e455032@.Control.Stream.EnableSelected) [COP(@a33d8fac@[7+@3992ee42@*3],@0e455032@.Status.Stream.Enabled,1) ,COP(@a33d8fac@[8+@3992ee42@*3],@0e455032@.Status.Stream.Configured,1) ,OTU(@0e455032@.Control.Stream.EnableSelected) OTU(@0e455032@.Control.Stream.DisableSelected) ] ,XIC(@0e455032@.Control.Stream.DisableSelected) [COP(@a33d8fac@[55+@3992ee42@*3],@0e455032@.Status.Stream.Enabled,1) ,COP(@a33d8fac@[56+@3992ee42@*3],@0e455032@.Status.Stream.Configured,1) ,OTU(@0e455032@.Control.Stream.EnableSelected) OTU(@0e455032@.Control.Stream.DisableSelected) ] ] ,[OTU(@0e455032@.Control.Stream.SetSelectedToActive) ,COP(@a33d8fac@[103+@3992ee42@*2],@64bd79af@,1) ,[XIC(@64bd79af@.8) OTL(@88140ee3@.0) ,XIO(@64bd79af@.8) OTU(@88140ee3@.0) ] ,[XIC(@64bd79af@.9) OTL(@88140ee3@.1) ,XIO(@64bd79af@.9) OTU(@88140ee3@.1) ] ,[XIC(@64bd79af@.10) OTL(@88140ee3@.2) ,XIO(@64bd79af@.10) OTU(@88140ee3@.2) ] ,[XIC(@64bd79af@.11) OTL(@88140ee3@.3) ,XIO(@64bd79af@.11) OTU(@88140ee3@.3) ] ,MVM(@64bd79af@,16#000F,@a9dcfd1c@) ADD(@a9dcfd1c@,1,@0e455032@.Status.Stream.Active) ,COP(@88140ee3@,@0e455032@.Status.Stream.EnableAlarm,1) ] ,[XIC(@0e455032@.Control.ResetAccumulators.ResetAccumulator1) OTU(@0e455032@.Control.ResetAccumulators.ResetAccumulator1) OTU(@0ec75abb@.Util.Buffer.MeterSignals[1+@3992ee42@*2].4) ,XIC(@0e455032@.Control.ResetAccumulators.ResetAccumulator2) OTU(@0e455032@.Control.ResetAccumulators.ResetAccumulator2) OTU(@0ec75abb@.Util.Buffer.MeterSignals[1+@3992ee42@*2].5) ,XIC(@0e455032@.Control.ResetAccumulators.ResetAccumulator3) OTU(@0e455032@.Control.ResetAccumulators.ResetAccumulator3) OTU(@0ec75abb@.Util.Buffer.MeterSignals[1+@3992ee42@*2].6) ,XIC(@0e455032@.Control.ResetAccumulators.ResetAccumulator4) OTU(@0e455032@.Control.ResetAccumulators.ResetAccumulator4) OTU(@0ec75abb@.Util.Buffer.MeterSignals[1+@3992ee42@*2].7) ,XIC(@0e455032@.Archive.Write.Daily) OTU(@0e455032@.Archive.Write.Daily) OTU(@0ec75abb@.Util.Buffer.MeterSignals[1+@3992ee42@*2].8) ,XIC(@0e455032@.Archive.Write.Hourly) OTU(@0e455032@.Archive.Write.Hourly) OTU(@0ec75abb@.Util.Buffer.MeterSignals[1+@3992ee42@*2].9) ] ,OTU(@0ec75abb@.Util.Block.InterruptPending.EnableDisable) OTL(@0ec75abb@.Util.Block.InterruptComplete.EnableDisable) OTU(@0ec75abb@.Util.Block.InterruptPending.Now) ];
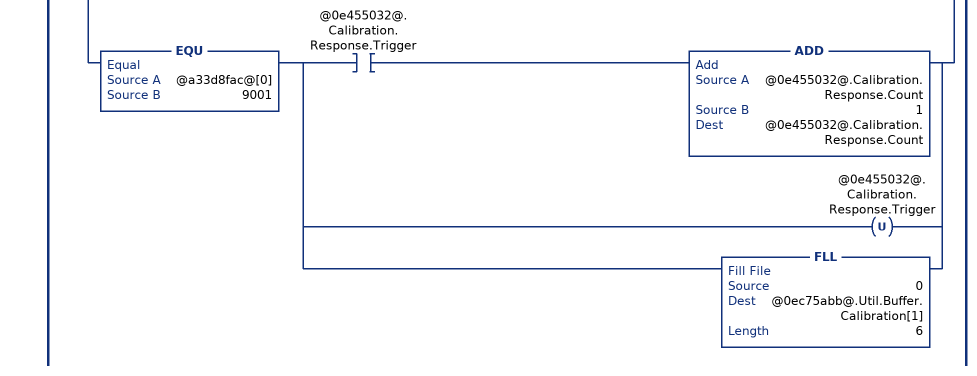
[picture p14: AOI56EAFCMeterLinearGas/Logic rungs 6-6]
   // Meter transmitter calibration.
   6: XIC(@54f1224f@)[EQU(@a33d8fac@[0],9000) ,EQU(@a33d8fac@[0],9001) ][MVM(@a33d8fac@[3],16#0F00,@2aaa9bff@) ,DIV(@2aaa9bff@,16#100,@2aaa9bff@) ]EQU(@2aaa9bff@,@3992ee42@)XIO(@a33d8fac@[3].14)[EQU(@a33d8fac@[0],9000) [XIO(@eecda6e6@) ADD(@0e455032@.Calibration.Request.Count,1,@0e455032@.Calibration.Request.Count) ,OTL(@eecda6e6@) [COP(@a33d8fac@[3],@bc90d670@,1) ,MVM(@bc90d670@,16#000F,@20c16291@) ] ,[EQU(@20c16291@,0) [OTL(@0e455032@.Calibration.Request.ProcessVariable.PulseFrequency) ,OTU(@0e455032@.Calibration.Request.ProcessVariable.Temperature) ,OTU(@0e455032@.Calibration.Request.ProcessVariable.Pressure) ] ,EQU(@20c16291@,1) [OTL(@0e455032@.Calibration.Request.ProcessVariable.Temperature) ,OTU(@0e455032@.Calibration.Request.ProcessVariable.PulseFrequency) ,OTU(@0e455032@.Calibration.Request.ProcessVariable.Pressure) ] ,EQU(@20c16291@,2) [OTL(@0e455032@.Calibration.Request.ProcessVariable.Pressure) ,OTU(@0e455032@.Calibration.Request.ProcessVariable.PulseFrequency) ,OTU(@0e455032@.Calibration.Request.ProcessVariable.Temperature) ] ] ,[[XIC(@a33d8fac@[5].2) [OTL(@0e455032@.Calibration.Request.ActionType.ZeroShift) ,COP(@a33d8fac@[6],@0e455032@.Calibration.Request.Value.ZeroShift.Applied,2) ] ,XIO(@a33d8fac@[5].2) [OTU(@0e455032@.Calibration.Request.ActionType.ZeroShift) ,FLL(0,@0e455032@.Calibration.Request.Value.ZeroShift.Applied,2) ] ] ,[XIC(@a33d8fac@[5].3) [OTL(@0e455032@.Calibration.Request.ActionType.SetZero) ,COP(@a33d8fac@[10],@0e455032@.Calibration.Request.Value.SetZero.Applied,2) ] ,XIO(@a33d8fac@[5].3) [OTU(@0e455032@.Calibration.Request.ActionType.SetZero) ,FLL(0,@0e455032@.Calibration.Request.Value.SetZero.Applied,2) ] ] ,[XIC(@a33d8fac@[5].4) [OTL(@0e455032@.Calibration.Request.ActionType.SetSpan) ,COP(@a33d8fac@[14],@0e455032@.Calibration.Request.Value.SetSpan.Applied,2) ] ,XIO(@a33d8fac@[5].4) [OTU(@0e455032@.Calibration.Request.ActionType.SetSpan) ,FLL(0,@0e455032@.Calibration.Request.Value.SetSpan.Applied,2) ] ] ,[XIC(@a33d8fac@[5].5) [OTL(@0e455032@.Calibration.Request.ActionType.SetMid1) ,COP(@a33d8fac@[18],@0e455032@.Calibration.Request.Value.SetMid1.Applied,2) ] ,XIO(@a33d8fac@[5].5) [OTU(@0e455032@.Calibration.Request.ActionType.SetMid1) ,FLL(0,@0e455032@.Calibration.Request.Value.SetMid1.Applied,2) ] ] ,[XIC(@a33d8fac@[5].6) [OTL(@0e455032@.Calibration.Request.ActionType.SetMid2) ,COP(@a33d8fac@[22],@0e455032@.Calibration.Request.Value.SetMid2.Applied,2) ] ,XIO(@a33d8fac@[5].6) [OTU(@0e455032@.Calibration.Request.ActionType.SetMid2) ,FLL(0,@0e455032@.Calibration.Request.Value.SetMid2.Applied,2) ] ] ,[XIC(@a33d8fac@[5].7) [OTL(@0e455032@.Calibration.Request.ActionType.SetMid3) ,COP(@a33d8fac@[26],@0e455032@.Calibration.Request.Value.SetMid3.Applied,2) ] ,XIO(@a33d8fac@[5].7) [OTU(@0e455032@.Calibration.Request.ActionType.SetMid3) ,FLL(0,@0e455032@.Calibration.Request.Value.SetMid3.Applied,2) ] ] ] ] ,EQU(@a33d8fac@[0],9001) [XIC(@0e455032@.Calibration.Response.Trigger) ADD(@0e455032@.Calibration.Response.Count,1,@0e455032@.Calibration.Response.Count) ,OTU(@0e455032@.Calibration.Response.Trigger) ,FLL(0,@0ec75abb@.Util.Buffer.Calibration[1],6) ] ];
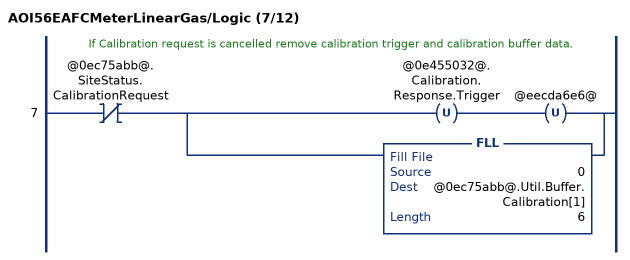
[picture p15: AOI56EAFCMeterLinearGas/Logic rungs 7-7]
   // If Calibration request is cancelled remove calibration trigger and calibration buffer data.
   7: XIO(@0ec75abb@.SiteStatus.CalibrationRequest)[OTU(@0e455032@.Calibration.Response.Trigger) OTU(@eecda6e6@) ,FLL(0,@0ec75abb@.Util.Buffer.Calibration[1],6) ];
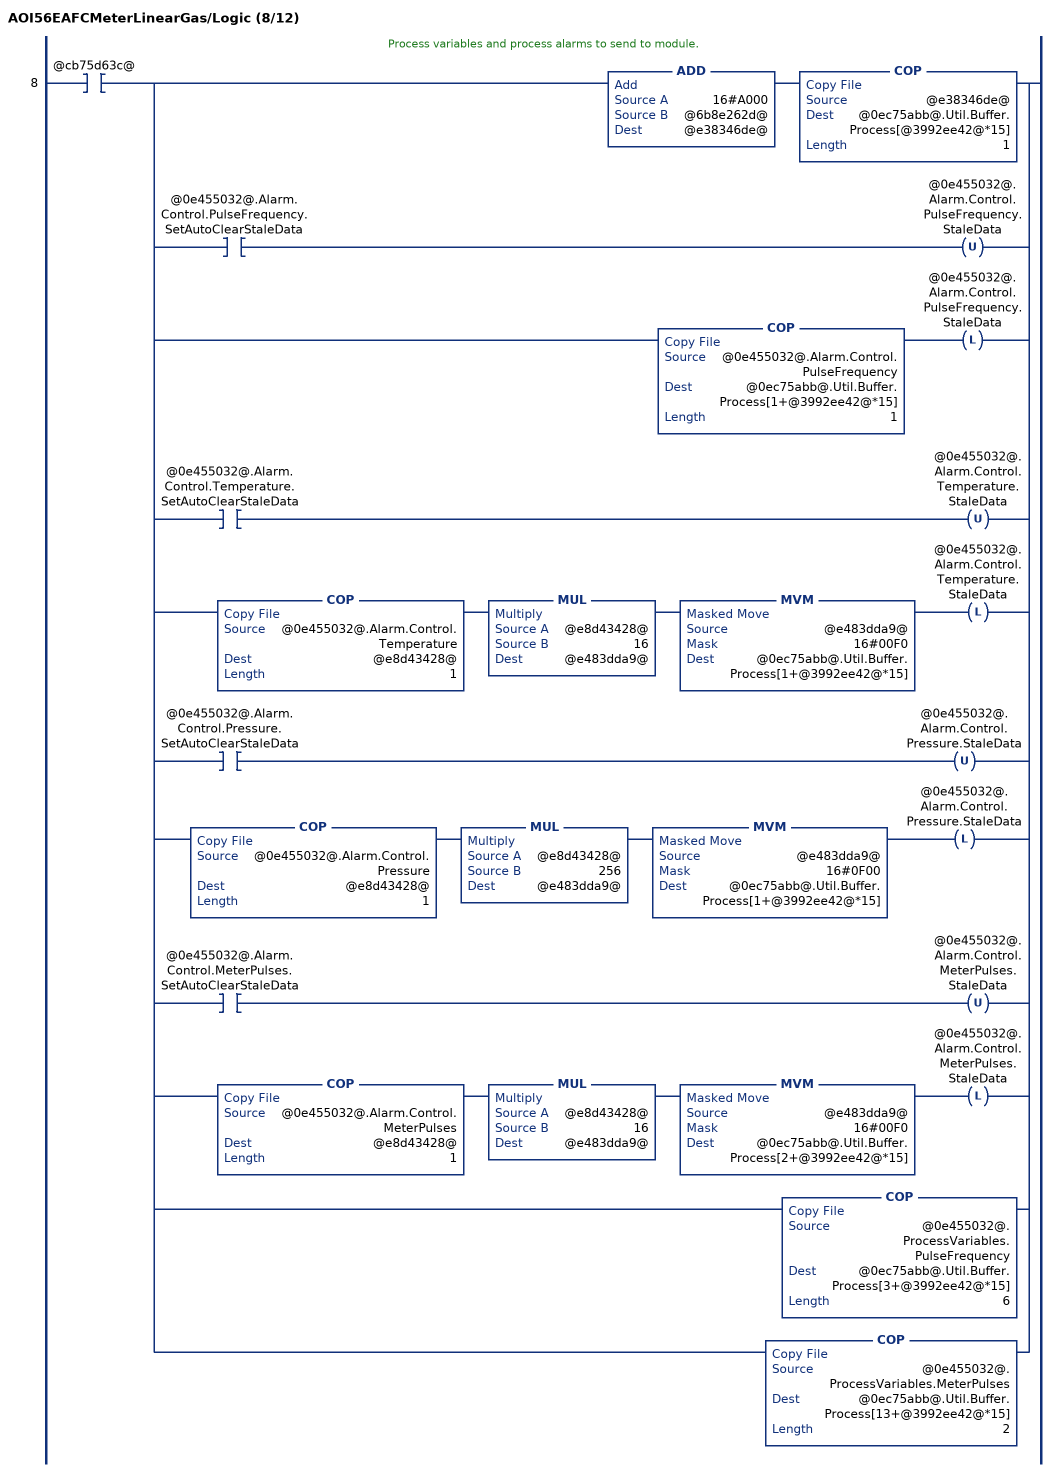
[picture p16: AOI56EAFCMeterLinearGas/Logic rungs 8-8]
   // Process variables and process alarms to send to module.
   8: XIC(@cb75d63c@)[ADD(16#A000,@6b8e262d@,@e38346de@) COP(@e38346de@,@0ec75abb@.Util.Buffer.Process[@3992ee42@*15],1) ,[XIC(@0e455032@.Alarm.Control.PulseFrequency.SetAutoClearStaleData) OTU(@0e455032@.Alarm.Control.PulseFrequency.StaleData) ,COP(@0e455032@.Alarm.Control.PulseFrequency,@0ec75abb@.Util.Buffer.Process[1+@3992ee42@*15],1) OTL(@0e455032@.Alarm.Control.PulseFrequency.StaleData) ] ,[XIC(@0e455032@.Alarm.Control.Temperature.SetAutoClearStaleData) OTU(@0e455032@.Alarm.Control.Temperature.StaleData) ,COP(@0e455032@.Alarm.Control.Temperature,@e8d43428@,1) MUL(@e8d43428@,16,@e483dda9@) MVM(@e483dda9@,16#00F0,@0ec75abb@.Util.Buffer.Process[1+@3992ee42@*15]) OTL(@0e455032@.Alarm.Control.Temperature.StaleData) ] ,[XIC(@0e455032@.Alarm.Control.Pressure.SetAutoClearStaleData) OTU(@0e455032@.Alarm.Control.Pressure.StaleData) ,COP(@0e455032@.Alarm.Control.Pressure,@e8d43428@,1) MUL(@e8d43428@,256,@e483dda9@) MVM(@e483dda9@,16#0F00,@0ec75abb@.Util.Buffer.Process[1+@3992ee42@*15]) OTL(@0e455032@.Alarm.Control.Pressure.StaleData) ] ,[XIC(@0e455032@.Alarm.Control.MeterPulses.SetAutoClearStaleData) OTU(@0e455032@.Alarm.Control.MeterPulses.StaleData) ,COP(@0e455032@.Alarm.Control.MeterPulses,@e8d43428@,1) MUL(@e8d43428@,16,@e483dda9@) MVM(@e483dda9@,16#00F0,@0ec75abb@.Util.Buffer.Process[2+@3992ee42@*15]) OTL(@0e455032@.Alarm.Control.MeterPulses.StaleData) ] ,[COP(@0e455032@.ProcessVariables.PulseFrequency,@0ec75abb@.Util.Buffer.Process[3+@3992ee42@*15],6) ,COP(@0e455032@.ProcessVariables.MeterPulses,@0ec75abb@.Util.Buffer.Process[13+@3992ee42@*15],2) ] ];
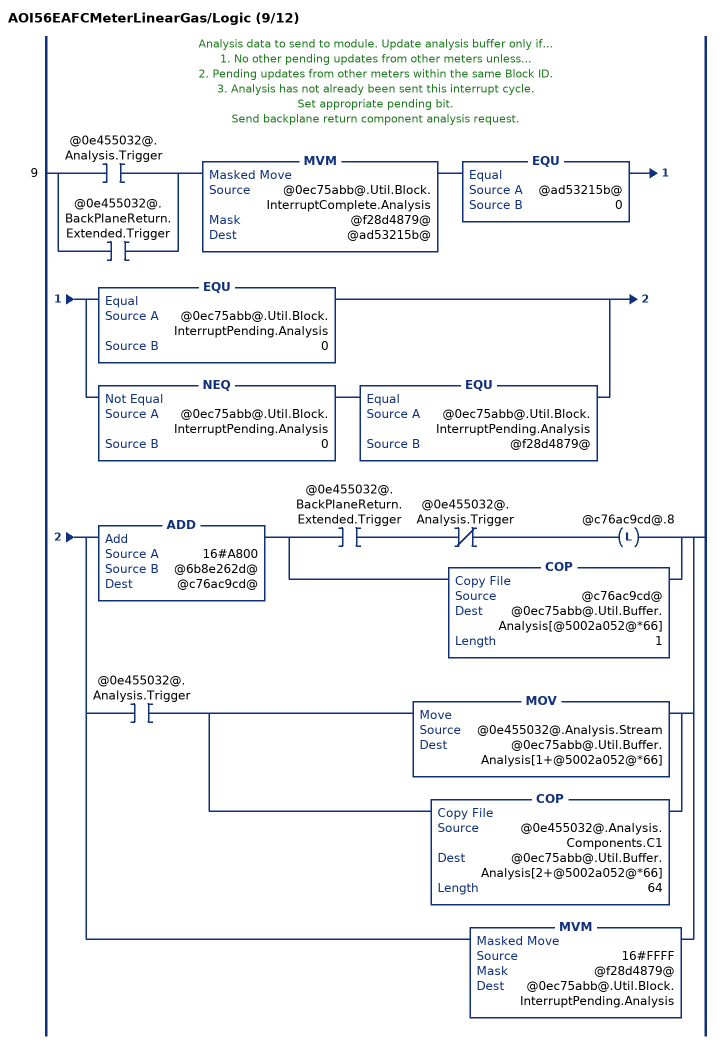
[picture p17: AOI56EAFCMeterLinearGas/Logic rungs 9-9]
   // Analysis data to send to module. Update analysis buffer only if...
   // 1. No other pending updates from other meters unless...
   // 2. Pending updates from other meters within the same Block ID.
   // 3. Analysis has not already been sent this interrupt cycle.
   // Set appropriate pending bit.
   // Send backplane return component analysis request.
   9: [XIC(@0e455032@.Analysis.Trigger) ,XIC(@0e455032@.BackPlaneReturn.Extended.Trigger) ]MVM(@0ec75abb@.Util.Block.InterruptComplete.Analysis,@f28d4879@,@ad53215b@)EQU(@ad53215b@,0)[EQU(@0ec75abb@.Util.Block.InterruptPending.Analysis,0) ,NEQ(@0ec75abb@.Util.Block.InterruptPending.Analysis,0) EQU(@0ec75abb@.Util.Block.InterruptPending.Analysis,@f28d4879@) ][ADD(16#A800,@6b8e262d@,@c76ac9cd@) [XIC(@0e455032@.BackPlaneReturn.Extended.Trigger) XIO(@0e455032@.Analysis.Trigger) OTL(@c76ac9cd@.8) ,COP(@c76ac9cd@,@0ec75abb@.Util.Buffer.Analysis[@5002a052@*66],1) ] ,XIC(@0e455032@.Analysis.Trigger) [MOV(@0e455032@.Analysis.Stream,@0ec75abb@.Util.Buffer.Analysis[1+@5002a052@*66]) ,COP(@0e455032@.Analysis.Components.C1,@0ec75abb@.Util.Buffer.Analysis[2+@5002a052@*66],64) ] ,MVM(16#FFFF,@f28d4879@,@0ec75abb@.Util.Block.InterruptPending.Analysis) ];
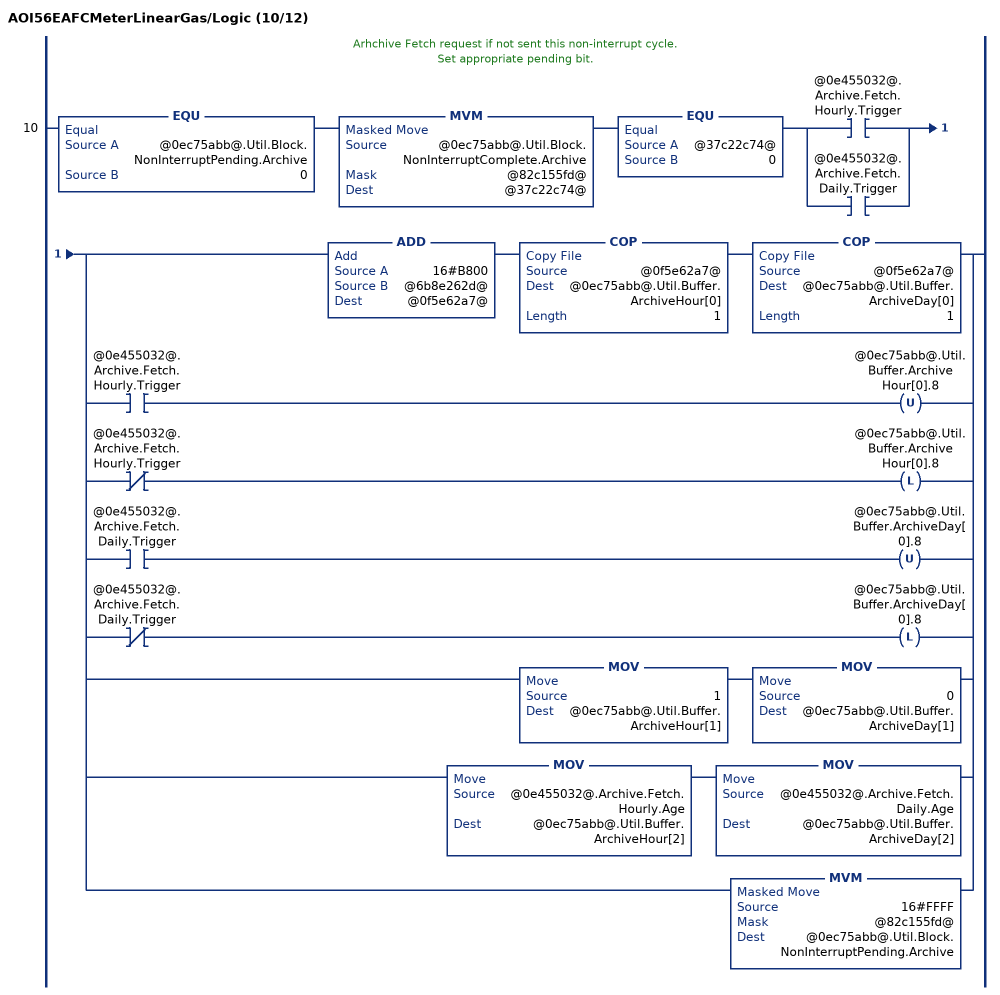
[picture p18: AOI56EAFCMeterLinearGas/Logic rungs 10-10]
   // Arhchive Fetch request if not sent this non-interrupt cycle.
   // Set appropriate pending bit.
   10: EQU(@0ec75abb@.Util.Block.NonInterruptPending.Archive,0)MVM(@0ec75abb@.Util.Block.NonInterruptComplete.Archive,@82c155fd@,@37c22c74@)EQU(@37c22c74@,0)[XIC(@0e455032@.Archive.Fetch.Hourly.Trigger) ,XIC(@0e455032@.Archive.Fetch.Daily.Trigger) ][ADD(16#B800,@6b8e262d@,@0f5e62a7@) COP(@0f5e62a7@,@0ec75abb@.Util.Buffer.ArchiveHour[0],1) COP(@0f5e62a7@,@0ec75abb@.Util.Buffer.ArchiveDay[0],1) ,[XIC(@0e455032@.Archive.Fetch.Hourly.Trigger) OTU(@0ec75abb@.Util.Buffer.ArchiveHour[0].8) ,XIO(@0e455032@.Archive.Fetch.Hourly.Trigger) OTL(@0ec75abb@.Util.Buffer.ArchiveHour[0].8) ] ,[XIC(@0e455032@.Archive.Fetch.Daily.Trigger) OTU(@0ec75abb@.Util.Buffer.ArchiveDay[0].8) ,XIO(@0e455032@.Archive.Fetch.Daily.Trigger) OTL(@0ec75abb@.Util.Buffer.ArchiveDay[0].8) ] ,MOV(1,@0ec75abb@.Util.Buffer.ArchiveHour[1]) MOV(0,@0ec75abb@.Util.Buffer.ArchiveDay[1]) ,MOV(@0e455032@.Archive.Fetch.Hourly.Age,@0ec75abb@.Util.Buffer.ArchiveHour[2]) MOV(@0e455032@.Archive.Fetch.Daily.Age,@0ec75abb@.Util.Buffer.ArchiveDay[2]) ,MVM(16#FFFF,@82c155fd@,@0ec75abb@.Util.Block.NonInterruptPending.Archive) ];
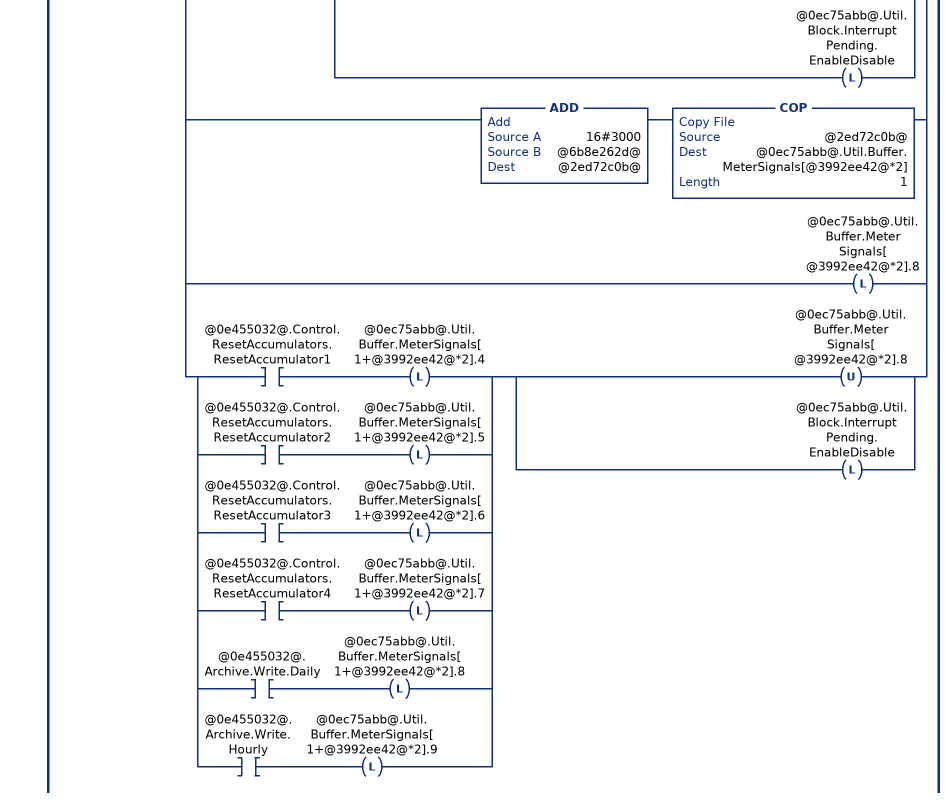
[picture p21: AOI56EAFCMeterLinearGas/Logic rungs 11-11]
   // Meter Enable.
   // Meter Disable.
   // Stream Select.
   // Stream Enable.
   // Stream Disable.
   // Set pending bit if not set this interrupt cycle.
   11: XIO(@0ec75abb@.Util.Block.InterruptComplete.EnableDisable)[LIM(1,@0e455032@.Control.Stream.Selected,16) CPT(@cc31c595@,2**(@0e455032@.Control.Stream.Selected-1)) ,[XIC(@0e455032@.Control.Meter.Enable) MVM(16#FFFF,@82c155fd@,@0ec75abb@.Util.Buffer.MeterEnableDisable[1]) MVM(16#0000,@82c155fd@,@0ec75abb@.Util.Buffer.MeterEnableDisable[3]) ,XIC(@0e455032@.Control.Meter.Disable) MVM(16#FFFF,@82c155fd@,@0ec75abb@.Util.Buffer.MeterEnableDisable[3]) MVM(16#0000,@82c155fd@,@0ec75abb@.Util.Buffer.MeterEnableDisable[1]) ] OTL(@0ec75abb@.Util.Block.InterruptPending.EnableDisable) ,[ADD(16#CC00,@6b8e262d@,@4102ecba@) COP(@4102ecba@,@0ec75abb@.Util.Buffer.StreamEnable[@3992ee42@*3],1) ,XIO(@0e455032@.Control.Stream.EnableSelected) OTL(@0ec75abb@.Util.Buffer.StreamEnable[@3992ee42@*3].8) ,XIC(@0e455032@.Control.Stream.EnableSelected) [OTU(@0ec75abb@.Util.Buffer.StreamEnable[@3992ee42@*3].8) ,COP(@cc31c595@,@0ec75abb@.Util.Buffer.StreamEnable[1+@3992ee42@*3],1) ,OTL(@0ec75abb@.Util.Block.InterruptPending.EnableDisable) ] ] ,[ADD(16#C800,@6b8e262d@,@3449dfe4@) COP(@3449dfe4@,@0ec75abb@.Util.Buffer.StreamDisable[@3992ee42@*3],1) ,XIO(@0e455032@.Control.Stream.DisableSelected) OTL(@0ec75abb@.Util.Buffer.StreamDisable[@3992ee42@*3].8) ,XIC(@0e455032@.Control.Stream.DisableSelected) [OTU(@0ec75abb@.Util.Buffer.StreamDisable[@3992ee42@*3].8) ,COP(@cc31c595@,@0ec75abb@.Util.Buffer.StreamDisable[1+@3992ee42@*3],1) ,OTL(@0ec75abb@.Util.Block.InterruptPending.EnableDisable) ] ] ,[ADD(16#3C00,@6b8e262d@,@9c0a19c1@) COP(@9c0a19c1@,@0ec75abb@.Util.Buffer.StreamSelect[@3992ee42@*2],1) ,XIO(@0e455032@.Control.Stream.SetSelectedToActive) OTL(@0ec75abb@.Util.Buffer.StreamSelect[@3992ee42@*2].8) ,XIC(@0e455032@.Control.Stream.SetSelectedToActive) [OTU(@0ec75abb@.Util.Buffer.StreamSelect[@3992ee42@*2].8) ,MOV(@0e455032@.Control.Stream.Selected,@0ec75abb@.Util.Buffer.StreamSelect[1+@3992ee42@*2]) ,OTL(@0ec75abb@.Util.Block.InterruptPending.EnableDisable) ] ] ,[ADD(16#3000,@6b8e262d@,@2ed72c0b@) COP(@2ed72c0b@,@0ec75abb@.Util.Buffer.MeterSignals[@3992ee42@*2],1) ,OTL(@0ec75abb@.Util.Buffer.MeterSignals[@3992ee42@*2].8) ,[XIC(@0e455032@.Control.ResetAccumulators.ResetAccumulator1) OTL(@0ec75abb@.Util.Buffer.MeterSignals[1+@3992ee42@*2].4) ,XIC(@0e455032@.Control.ResetAccumulators.ResetAccumulator2) OTL(@0ec75abb@.Util.Buffer.MeterSignals[1+@3992ee42@*2].5) ,XIC(@0e455032@.Control.ResetAccumulators.ResetAccumulator3) OTL(@0ec75abb@.Util.Buffer.MeterSignals[1+@3992ee42@*2].6) ,XIC(@0e455032@.Control.ResetAccumulators.ResetAccumulator4) OTL(@0ec75abb@.Util.Buffer.MeterSignals[1+@3992ee42@*2].7) ,XIC(@0e455032@.Archive.Write.Daily) OTL(@0ec75abb@.Util.Buffer.MeterSignals[1+@3992ee42@*2].8) ,XIC(@0e455032@.Archive.Write.Hourly) OTL(@0ec75abb@.Util.Buffer.MeterSignals[1+@3992ee42@*2].9) ] [OTU(@0ec75abb@.Util.Buffer.MeterSignals[@3992ee42@*2].8) ,OTL(@0ec75abb@.Util.Block.InterruptPending.EnableDisable) ] ] ];
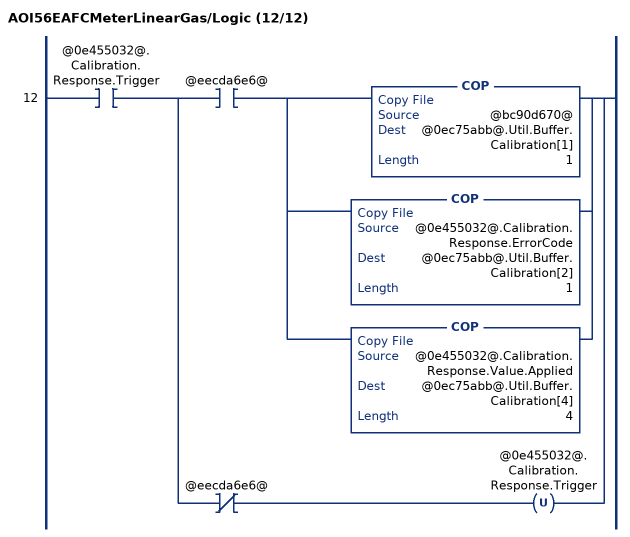
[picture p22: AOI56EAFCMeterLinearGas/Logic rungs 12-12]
   12: XIC(@0e455032@.Calibration.Response.Trigger)[XIC(@eecda6e6@) [COP(@bc90d670@,@0ec75abb@.Util.Buffer.Calibration[1],1) ,COP(@0e455032@.Calibration.Response.ErrorCode,@0ec75abb@.Util.Buffer.Calibration[2],1) ,COP(@0e455032@.Calibration.Response.Value.Applied,@0ec75abb@.Util.Buffer.Calibration[4],4) ] ,XIO(@eecda6e6@) OTU(@0e455032@.Calibration.Response.Trigger) ];
END_ROUTINE

ROUTINE Prescan   (* ladder *)
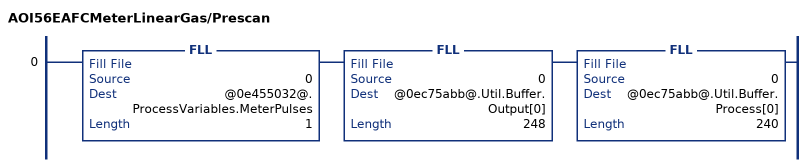
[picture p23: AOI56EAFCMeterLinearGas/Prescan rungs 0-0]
   0: FLL(0,@0e455032@.ProcessVariables.MeterPulses,1)FLL(0,@0ec75abb@.Util.Buffer.Output[0],248)FLL(0,@0ec75abb@.Util.Buffer.Process[0],240);
END_ROUTINE
END_ADD_ON_INSTRUCTION

VAR_GLOBAL   (* controller tags *)
   AFC : AFCEModuleDef;
   AOI56EAFCMeter03LinearGas : AOI56EAFCMeterLinearGas;
   AFCMeter03LinearGas : AFCEMeterLinearGas;
   Local:1:I : AB:1756_MODULE_INT_500Bytes:I:0;
END_VAR

PROGRAM MainProgram

ROUTINE MainRoutine   (* ladder *)
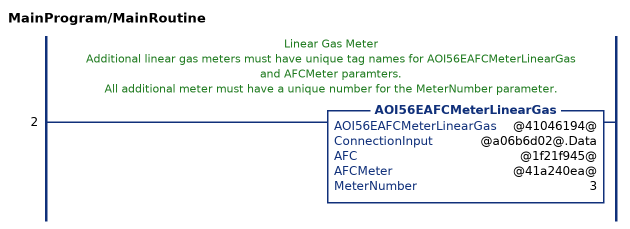
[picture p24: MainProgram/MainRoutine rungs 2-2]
   // Linear Gas Meter
   // Additional linear gas meters must have unique tag names for AOI56EAFCMeterLinearGas and AFCMeter paramters.
   // All additional meter must have a unique number for the MeterNumber parameter.
   2: AOI56EAFCMeterLinearGas(@41046194@,@a06b6d02@.Data,@1f21f945@,@41a240ea@,3);
END_ROUTINE
END_PROGRAM
